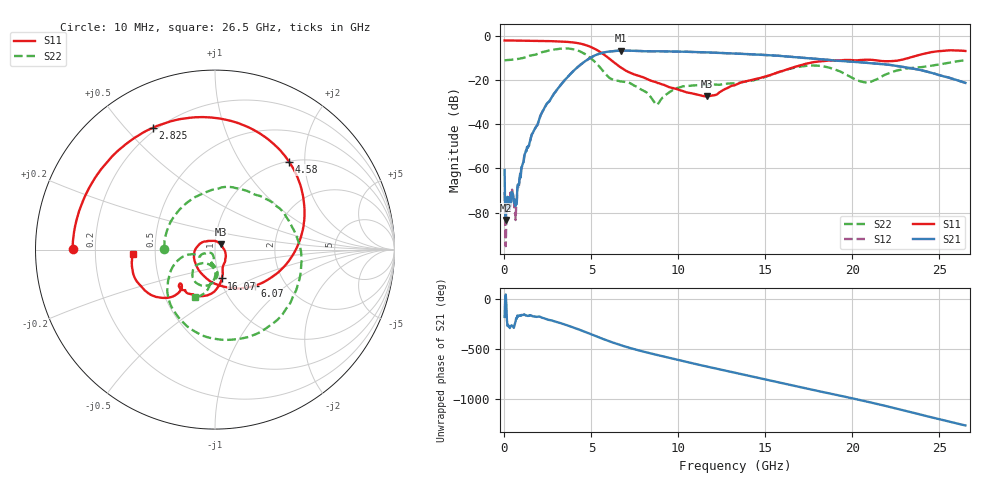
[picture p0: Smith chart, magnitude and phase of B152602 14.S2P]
!  2-Port S-parameters saved by WinCal
! VAR MeasName=S-Parameters (CALIBRATED_DATA) read from VNA (N5242A)
! VAR MeasDate=2016-1-5 16:27:21
! VAR NAME=B152602 14
! VAR FILENAME=B152602 14.S2P
! VAR DATE=2016-1-5 16:27:21
! VAR PHYS_PORTS=1,2
# Hz S DB R 50
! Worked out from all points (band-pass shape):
!   801 points, 10 MHz to 26.5 GHz, reference 50 ohm
!   highest |S21| = -6.63 dB at 6.699 GHz (marker M1); lowest = -83.4 dB at 76.22 MHz (marker M2)
!   |S21| within 3 dB of the highest: 4.995 GHz to 16.79 GHz (11.79 GHz wide, 108 % of centre)
!   lowest |S11| = -27.4 dB at 11.67 GHz (marker M3), VSWR 1.09, Z = 53.2 + j3.07 ohm
!   |S11| at or under -10 dB: 5.99 GHz to 23.22 GHz (17.23 GHz wide, 118 % of centre)
!   |S22| runs from -31.2 to -5.6 dB; largest |S21 - S12| = 0.0029
!   S11 on the Smith chart (normalised r, x): 10 MHz: 0.12, +0.00; 2.825 GHz: 0.18, +0.60; 4.58 GHz: 1.01, +1.67; 6.07 GHz: 1.40, -0.62; 16.07 GHz: 1.02, -0.34; 26.5 GHz: 0.37, -0.02
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1e7  -2.01 179.7  -60.73 -177.5  -70.78 -6.3  -10.99 179.4
7.6225e7  -2.01 178.4  -83.41 47.2  -95.26 -109.6  -10.96 174.8
1.755625e8  -2.02 176.3  -72.90 91.8  -73.42 80.6  -10.88 167.4
6.7225e8  -2.07 166.2  -76.17 167.4  -77.77 175.4  -10.51 131.3
1.268275e9  -2.15 153.9  -52.18 -163.7  -52.21 -165.4  -9.45 90.4
2.824562e9  -2.36 117.0  -26.43 141.1  -26.43 141.1  -6.14 -14.0
3.685488e9  -2.70 89.3  -18.06 93.3  -18.08 93.3  -5.67 -70.0
4.447075e9  -3.60 56.5  -12.55 45.0  -12.57 45.1  -7.34 -118.2
4.579525e9  -3.88 49.8  -11.76 36.5  -11.77 36.5  -7.85 -125.8
5.341112e9  -6.46 6.3  -8.33 -16.4  -8.33 -16.3  -12.84 -161.9
6.069588e9  -10.49 -42.5  -6.98 -65.0  -6.98 -65.0  -19.13 -164.4
6.698725e9  -14.28 -88.0  -6.63 -102.1  -6.64 -102.1  -20.58 -154.8
8.851038e9  -21.35 154.6  -6.92 157.1  -6.91 157.0  -30.53 -116.9
1.027488e10  -24.99 120.4  -7.09 98.0  -7.10 97.9  -22.77 -101.6
1.16656e10  -27.37 42.4  -7.44 42.2  -7.44 42.3  -22.07 -103.6
1.3255e10  -22.24 -42.6  -7.92 -18.9  -7.91 -18.9  -21.39 -96.4
1.606956e10  -15.63 -76.8  -9.22 -127.6  -9.16 -127.6  -15.71 -88.5
1.769208e10  -11.95 -97.1  -10.21 171.1  -10.18 171.2  -13.37 -113.0
2.073842e10  -10.76 -129.8  -12.10 55.4  -12.05 55.3  -21.04 -115.7
2.209604e10  -11.43 -134.3  -13.06 0.3  -13.01 0.0  -16.88 -89.2
2.388411e10  -8.45 -134.6  -15.40 -76.7  -15.35 -77.1  -14.18 -98.2
2.65e10  -6.78 -176.8  -21.24 172.2  -21.26 172.0  -10.93 -112.7
